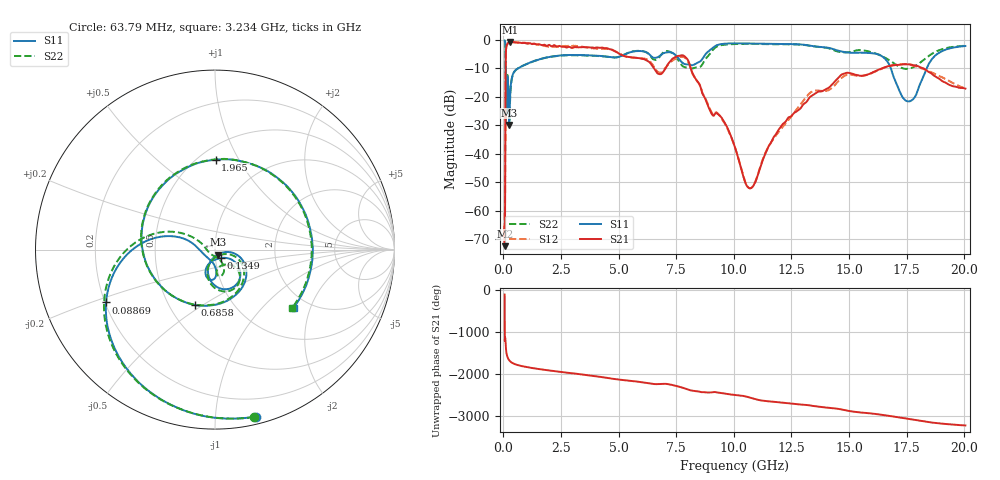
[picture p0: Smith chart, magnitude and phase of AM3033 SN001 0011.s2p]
# Hz S DB R 50
!freq MagS11 AngS11 MagS21 AngS21 MagS12 AngS12 MagS22 AngS22
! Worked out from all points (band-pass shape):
!   1601 points, 50 MHz to 20.05 GHz, reference 50 ohm
!   highest |S21| = -0.70 dB at 294.1 MHz (marker M1); lowest = -72.5 dB at 62.84 MHz (marker M2)
!   |S21| within 3 dB of the highest: 108.8 MHz to 4.778 GHz (4.669 GHz wide, 191 % of centre)
!   lowest |S11| = -29.9 dB at 250.4 MHz (marker M3), VSWR 1.07, Z = 51.4 - j2.92 ohm
!   |S11| at or under -10 dB: 94.46 MHz to 623.6 MHz (529.2 MHz wide, 147 % of centre); 16.82 GHz to 18.37 GHz (1.554 GHz wide, 8.83 % of centre)
!   |S22| runs from -29.5 to -0.2 dB; largest |S21 - S12| = 0.064
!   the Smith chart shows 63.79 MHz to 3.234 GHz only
!   S11 on the Smith chart (normalised r, x): 63.79 MHz: 0.06, -1.27; 88.69 MHz: 0.20, -0.22; 134.9 MHz: 1.06, -0.10; 685.8 MHz: 0.67, -0.46; 1.965 GHz: 0.60, +0.81; 3.234 GHz: 1.67, -1.54
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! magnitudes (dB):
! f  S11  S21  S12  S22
! 50 MHz  -0.2  -72.2  -60.8  -0.2
! 62.84 MHz  -0.4  -72.5  -68.3  -0.3
! 63.79 MHz  -0.4  -70.8  -67.6  -0.4
! 88.69 MHz  -3.4  -20.8  -20.8  -3.5
! 102.6 MHz  -23.5  -5.0  -5.0  -29.4
! 134.9 MHz  -24.9  -1.9  -1.9  -19.8
! 135.9 MHz  -24.2  -1.9  -1.9  -19.5
! 178.7 MHz  -12.9  -1.3  -1.4  -12.5
! 250.4 MHz  -29.9  -0.7  -0.8  -28.0
! 294.1 MHz  -18.8  -0.7  -0.7  -19.1
! 369.6 MHz  -13.2  -0.8  -0.7  -13.4
! 685.8 MHz  -9.7  -0.9  -1.0  -9.7
! 1.005 GHz  -8.5  -1.3  -1.1  -8.4
! 1.965 GHz  -6.0  -1.7  -2.3  -6.0
! 2.722 GHz  -5.3  -2.6  -2.2  -5.4
! 3.234 GHz  -5.3  -2.6  -2.2  -5.4
! 7.402 GHz  -4.8  -6.3  -6.9  -5.1
! 9.549 GHz  -1.3  -28.4  -28.6  -1.7
! 10.69 GHz  -1.2  -52.1  -52.1  -1.4
! 14.75 GHz  -4.2  -11.9  -12.9  -4.4
! 17.59 GHz  -21.6  -8.6  -8.6  -10.1
! 20.05 GHz  -2.1  -17.1  -17.0  -2.0
